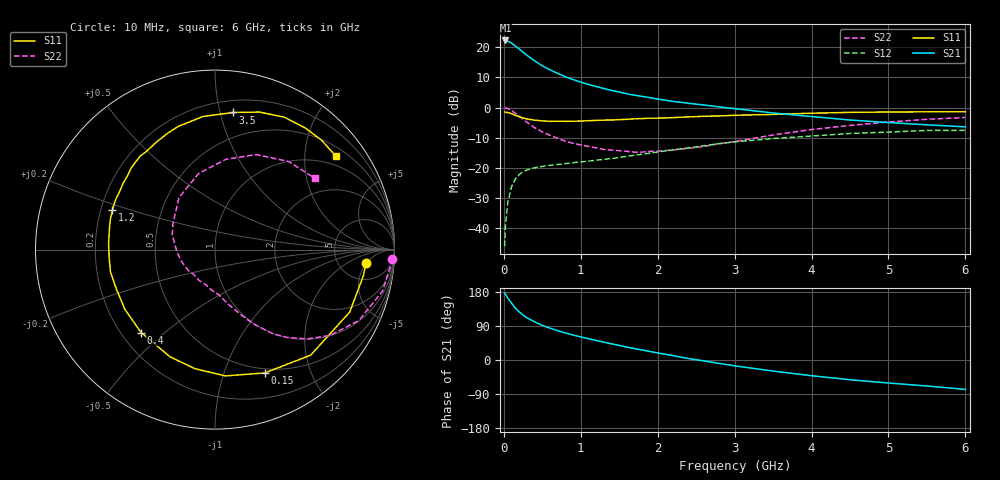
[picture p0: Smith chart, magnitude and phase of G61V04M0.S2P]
! SIEMENS Small Signal Semiconductors
! BFG193
! Si NPN RF Bipolar Junction Transistor in SOT223
! VCE = 1 V  IC = 4 mA
! Common Emitter S-Parameters:  August  1996
# GHz  S  MA  R  50
!  f  S11  S21  S12  S22
! GHz  MAG  ANG  MAG  ANG  MAG  ANG  MAG  ANG
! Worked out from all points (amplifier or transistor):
!   36 points, 10 MHz to 6 GHz, reference 50 ohm
!   highest |S21| = 22.2 dB at 20 MHz (marker M1)
!   |S21| within 3 dB of that: start of sweep to 207.7 MHz
!   unconditionally stable (mu >= 1): 1.151 GHz to 2.963 GHz
!   at 250 MHz: K = 0.30, MSG = 19.8 dB, |S12| = -21.2 dB
!   at 1.4 GHz: K = 1.10, MAG = 9.3 dB, |S12| = -16.9 dB
!   at 6 GHz: K = 0.97, MSG = 0.6 dB, |S12| = -7.5 dB
!   S11 on the Smith chart (normalised r, x): 10 MHz: 9, -5; 150 MHz: 0.45, -1.38; 400 MHz: 0.28, -0.42; 1.2 GHz: 0.25, +0.18; 3.5 GHz: 0.29, +1.10; 6 GHz: 0.73, +2.76
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0.01  0.8439 -5.0  12.8 176.6  0.0051 90.3  0.9895 -2.9
0.02  0.8396 -10.0  12.87 174.2  0.0106 87.2  0.9806 -5.6
0.05  0.8273 -24.9  12.57 163.3  0.0263 76.4  0.9617 -13.9
0.1  0.7937 -47.8  11.62 150.1  0.049 66.2  0.8941 -26.2
0.15  0.741 -68.0  10.4 136.6  0.066 55.5  0.801 -36.6
0.2  0.7061 -85.3  9.288 127.1  0.0779 49.2  0.7166 -44.0
0.25  0.6727 -99.6  8.216 118.3  0.0868 43.5  0.6333 -50.6
0.3  0.6475 -112.8  7.321 111.4  0.0928 39.5  0.5703 -55.4
0.4  0.6188 -131.7  5.931 100.7  0.1012 34.1  0.4657 -62.7
0.5  0.6024 -146.4  4.893 91.4  0.1064 30.4  0.3949 -67.8
0.6  0.5918 -158.2  4.208 84.0  0.1109 28.9  0.3475 -72.3
0.7  0.5954 -168.1  3.677 77.3  0.1146 28.0  0.3099 -76.9
0.9  0.5939 176.6  2.904 65.9  0.1225 27.1  0.2556 -84.5
1.1  0.6064 164.2  2.408 56.2  0.1301 26.9  0.2277 -94.1
1.2  0.6128 158.8  2.227 51.6  0.1344 27.3  0.2153 -99.1
1.6  0.6384 139.6  1.687 34.0  0.1564 26.7  0.1889 -122.6
2.2  0.6821 118.6  1.264 11.4  0.1999 22.4  0.199 -162.0
2.8  0.7274 100.4  1.026 -9.0  0.2526 13.9  0.2527 160.4
3.5  0.7707 82.4  0.814 -29.2  0.3073 -1.0  0.3523 124.8
4.5  0.833 62.3  0.622 -52.1  0.373 -20.7  0.5069 83.2
5.5  0.8509 45.8  0.518 -68.6  0.4182 -44.7  0.6395 50.2
6  0.8512 37.6  0.48 -77.6  0.4196 -58.3  0.6842 35.4
